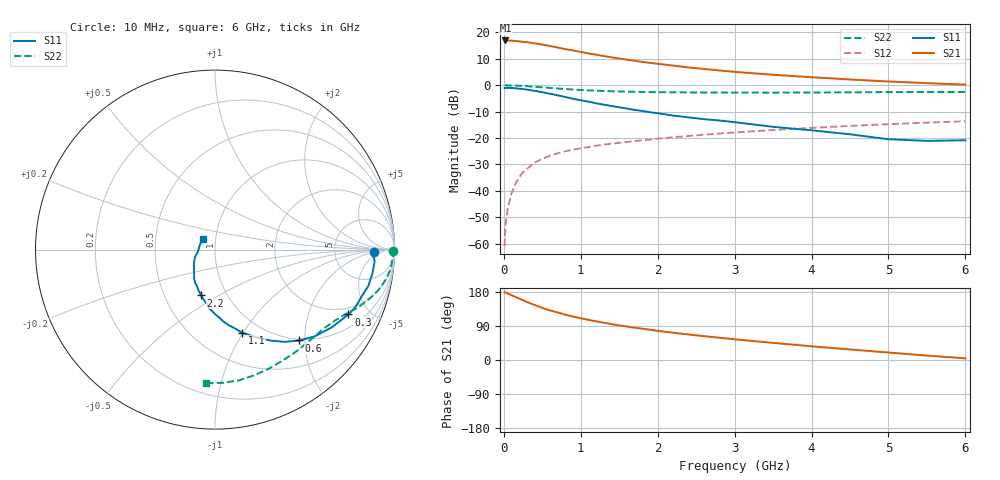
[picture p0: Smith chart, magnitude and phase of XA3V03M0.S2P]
! SIEMENS Discrete & RF Semiconductors
! BFY180
! Si NPN RF Bipolar Junction Transistor in MICRO-X
! VCE = 3 V  IC = 3 mA
! Common Emitter S-Parameters:  May  1997
# GHz  S  MA  R  50
!  f  S11  S21  S12  S22
! GHz  MAG  ANG  MAG  ANG  MAG  ANG  MAG  ANG
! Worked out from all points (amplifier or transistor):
!   36 points, 10 MHz to 6 GHz, reference 50 ohm
!   highest |S21| = 16.9 dB at 20 MHz (marker M1)
!   |S21| within 3 dB of that: start of sweep to 752.1 MHz
!   unconditionally stable (mu >= 1): 2.128 GHz to end of sweep
!   at 250 MHz: K = 0.16, MSG = 24.6 dB, |S12| = -32.9 dB
!   at 1.4 GHz: K = 0.83, MSG = 16.3 dB, |S12| = -22.1 dB
!   at 6 GHz: K = 1.08, MAG = 5.2 dB, |S12| = -13.6 dB
!   S11 on the Smith chart (normalised r, x): 10 MHz: 16, -2; 300 MHz: 1.62, -3.68; 600 MHz: 0.97, -1.88; 1.1 GHz: 0.82, -0.99; 2.2 GHz: 0.76, -0.42; 6 GHz: 0.87, +0.10
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0.01  0.8871 -0.8  6.955 178.9  0.0009 92.8  0.9921 -0.3
0.02  0.8822 -1.9  7.031 177.9  0.0022 83.7  0.9999 -0.8
0.05  0.8918 -4.2  6.96 175.5  0.0046 90.3  0.9924 -1.9
0.1  0.8869 -8.9  6.95 171.0  0.0091 86.4  0.9878 -3.9
0.2  0.8586 -17.5  6.766 161.9  0.0181 80.1  0.9778 -7.5
0.3  0.8266 -25.9  6.517 153.3  0.0261 75.2  0.9584 -11.0
0.4  0.782 -33.6  6.205 145.2  0.0343 71.3  0.9367 -14.0
0.5  0.7379 -40.8  5.881 137.7  0.0404 66.5  0.9117 -16.8
0.6  0.6901 -47.2  5.518 130.8  0.0465 64.2  0.8879 -19.1
0.8  0.5973 -58.2  4.813 119.5  0.0563 59.1  0.8476 -23.0
1  0.5189 -67.3  4.266 110.1  0.0641 55.5  0.8123 -26.2
1.1  0.4889 -71.8  3.999 106.0  0.0676 54.2  0.7993 -27.6
1.3  0.4283 -79.6  3.562 98.4  0.0752 52.0  0.7778 -30.4
1.5  0.3823 -86.0  3.207 91.3  0.0814 50.5  0.7622 -33.1
1.7  0.3405 -93.1  2.91 85.1  0.0878 49.1  0.7498 -35.6
2.2  0.2667 -106.8  2.352 71.9  0.1035 46.0  0.7341 -42.3
2.6  0.2279 -116.1  2.033 62.8  0.1156 43.5  0.7276 -47.5
3  0.1999 -125.4  1.79 54.6  0.1276 41.0  0.7255 -52.6
3.5  0.1632 -135.9  1.577 45.2  0.1417 37.8  0.7242 -59.1
4.5  0.1178 -160.2  1.284 27.8  0.1697 30.6  0.733 -72.5
5.5  0.0884 164.2  1.095 11.7  0.1961 22.8  0.7436 -86.8
6  0.0908 139.0  1.026 4.4  0.2081 18.6  0.7445 -94.0
